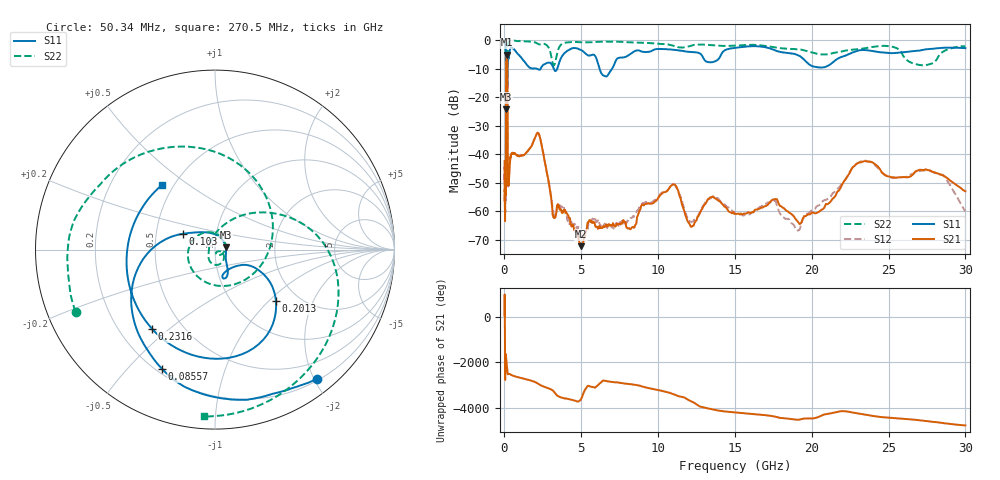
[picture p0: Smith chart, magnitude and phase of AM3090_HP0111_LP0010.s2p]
! Date/Time: Thu, Feb 28, 2019 2:00 PM
! Network Analyzer: Agilent Technologies E8364B Rev: A.07.50.67
! Sweep from 0.010 to 30.000 GHz, 1601 Points, Sweep Type: LOG
! Power Supply: 5.023 V, 0.002 A
# Hz S DB R 50
!freq MagS11 AngS11 MagS21 AngS21 MagS12 AngS12 MagS22 AngS22
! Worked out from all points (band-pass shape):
!   1601 points, 10 MHz to 30 GHz, reference 50 ohm
!   highest |S21| = -5.14 dB at 146.2 MHz (marker M1); lowest = -72.3 dB at 4.977 GHz (marker M2)
!   |S21| within 3 dB of the highest: 112.2 MHz to 185.5 MHz (73.31 MHz wide, 49.3 % of centre)
!   lowest |S11| = -24.2 dB at 109.9 MHz (marker M3), VSWR 1.13, Z = 56.4 + j1.43 ohm
!   |S11| at or under -10 dB: 2.058 GHz to 2.362 GHz (303.7 MHz wide, 13.7 % of centre); 3.205 GHz to 3.442 GHz (236.7 MHz wide, 7.12 % of centre); 6.184 GHz to 7.011 GHz (826.7 MHz wide, 12.5 % of centre)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
!   |S22| runs from -35.9 to -0.2 dB; largest |S21 - S12| = 0.0099
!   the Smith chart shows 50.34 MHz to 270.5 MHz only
!   S11 on the Smith chart (normalised r, x): 50.34 MHz: 0.23, -2.04; 85.57 MHz: 0.22, -0.63; 103 MHz: 0.69, +0.13; 201.3 MHz: 1.55, -1.10; 231.6 MHz: 0.34, -0.44; 270.5 MHz: 0.43, +0.40
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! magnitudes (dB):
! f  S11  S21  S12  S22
! 10 MHz  -0.3  -42.4  -49.1  -0.5
! 38.04 MHz  -0.5  -62.9  -60.8  -1.3
! 50.34 MHz  -0.8  -48.8  -53.6  -1.4
! 85.57 MHz  -2.8  -50.1  -51.1  -5.9
! 103 MHz  -14.1  -15.6  -15.6  -15.2
! 109.9 MHz  -24.2  -9.1  -9.1  -18.5
! 144.7 MHz  -16.9  -5.1  -5.1  -29.8
! 146.2 MHz  -17.0  -5.1  -5.1  -27.4
! 178.6 MHz  -15.1  -6.8  -6.7  -29.1
! 201.3 MHz  -7.1  -20.3  -20.3  -8.6
! 231.6 MHz  -5.0  -50.5  -50.9  -1.4
! 270.5 MHz  -6.6  -50.7  -51.1  -0.6
! 550.5 MHz  -3.0  -39.8  -39.6  -0.3
! 2.084 GHz  -10.0  -33.0  -33.0  -1.0
! 3.236 GHz  -10.4  -62.3  -61.4  -8.8
! 4.977 GHz  -3.5  -72.3  -67.2  -0.8
! 7.926 GHz  -5.8  -65.6  -64.3  -0.7
! 10.86 GHz  -3.3  -51.0  -50.9  -1.8
! 12.19 GHz  -4.2  -65.5  -63.8  -1.9
! 18.93 GHz  -5.0  -62.7  -66.0  -3.2
! 23.48 GHz  -3.5  -42.5  -42.2  -2.9
! 30 GHz  -2.8  -53.1  -60.2  -2.2
